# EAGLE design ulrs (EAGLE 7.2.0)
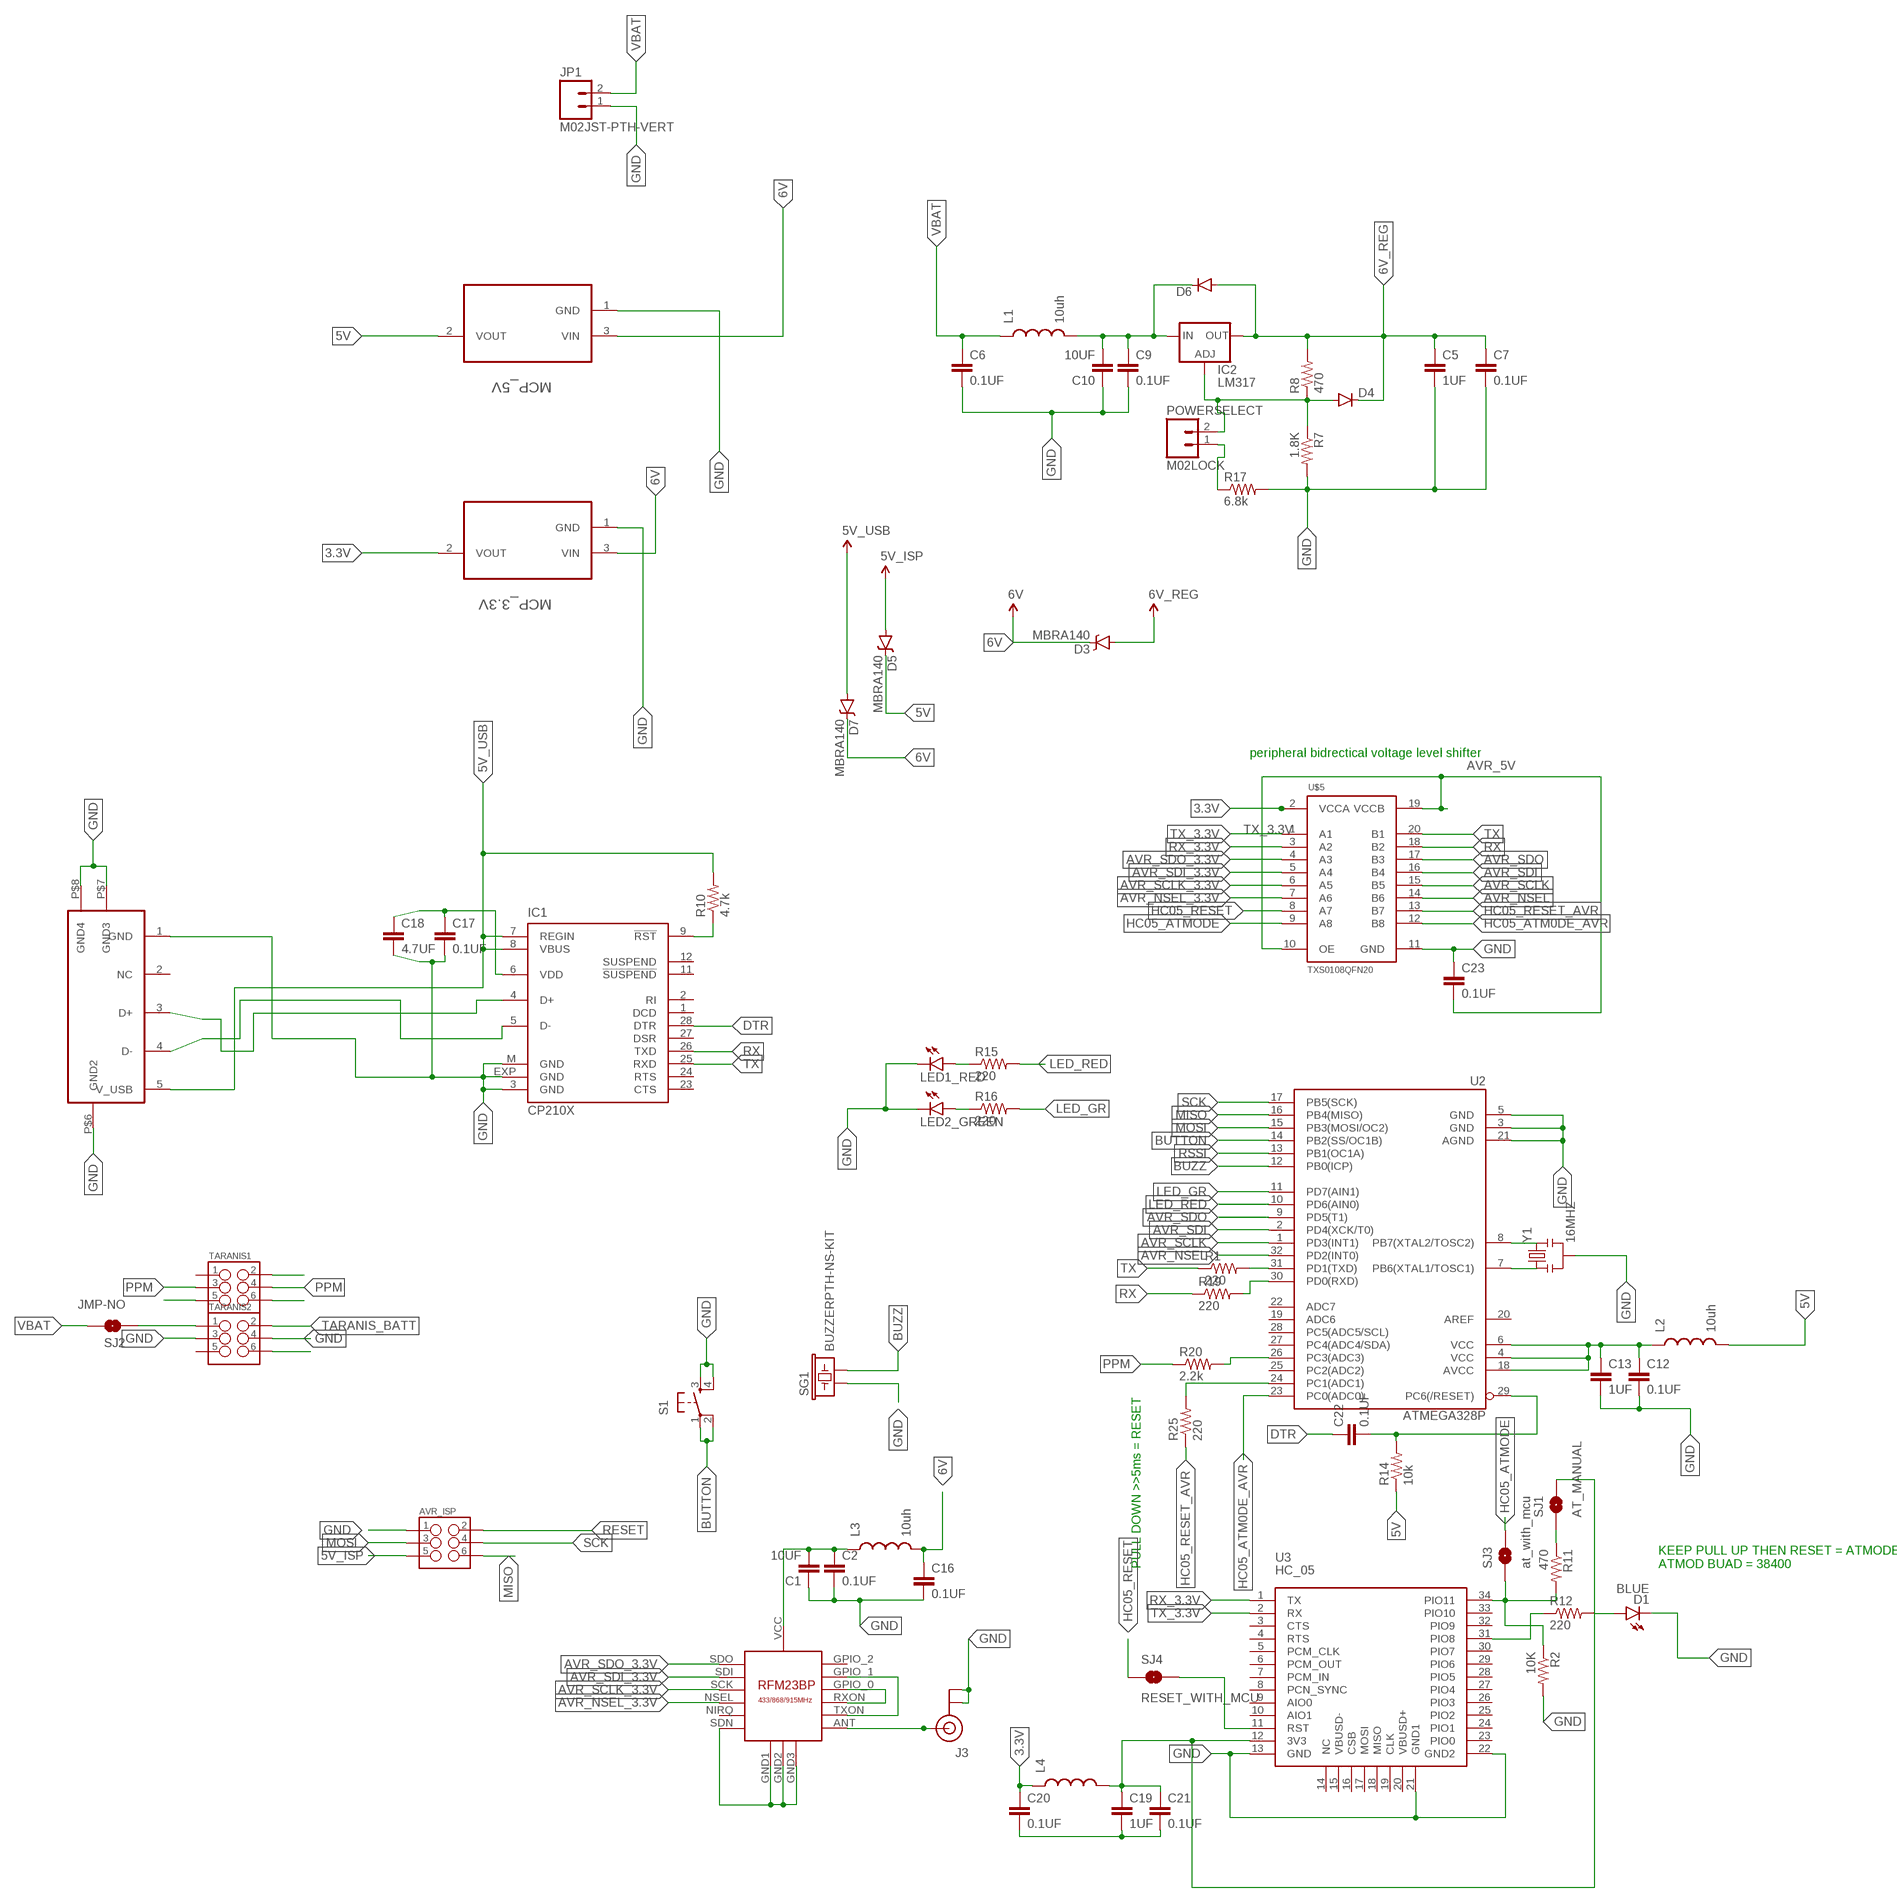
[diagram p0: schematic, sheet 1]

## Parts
AVR_ISP  M03X2FEMALE_SMD  [2X3_SMD]
C1  10UF  CAP1206  [1206]
C2  0.1UF  CAP0402-CAP  [0402-CAP]
C5  1UF  CAP0402-CAP  [0402-CAP]
C6  0.1UF  CAP0402-CAP  [0402-CAP]
C7  0.1UF  CAP0402-CAP  [0402-CAP]
C9  0.1UF  CAP0402-CAP  [0402-CAP]
C10  10UF  CAP1206  [1206]
C12  0.1UF  CAP0402-CAP  [0402-CAP]
C13  1UF  CAP0402-CAP  [0402-CAP]
C16  0.1UF  CAP0402-CAP  [0402-CAP]
C17  0.1UF  CAP0402-CAP  [0402-CAP]
C18  4.7UF  CAP0402-CAP  [0402-CAP]
C19  1UF  CAP0402-CAP  [0402-CAP]
C20  0.1UF  CAP0402-CAP  [0402-CAP]
C21  0.1UF  CAP0402-CAP  [0402-CAP]
C22  0.1UF  CAP0402-CAP  [0402-CAP]
C23  0.1UF  CAP0402-CAP  [0402-CAP]
D1  BLUE  LED-BLUE0603  [LED-0603]
D3  MBRA140  DIODE-SCHOTTKY-MBRA140  [SMA-DIODE]
D4  DIODESMA  [SMA-DIODE]
D5  MBRA140  DIODE-SCHOTTKY-MBRA140  [SMA-DIODE]
D6  DIODESMA  [SMA-DIODE]
D7  MBRA140  DIODE-SCHOTTKY-MBRA140  [SMA-DIODE]
IC1  CP210X  CP210X_USB_UART  [MLP28]
IC2  LM317  LM317MBSTT3  [SOT223]
J3  U.FL  [U.FL]
JP1  M02JST-PTH-VERT  [JST-2-PTH-VERT]
L1  10uh  INDUCTOR1007  [1007]
L2  10uh  INDUCTOR1007  [1007]
L3  10uh  INDUCTOR1007  [1007]
L4  INDUCTOR1007  [1007]
LED1_RED  LED3MM  [LED3MM]
LED2_GREEN  LED3MM  [LED3MM]
MCP_3.3V  MCP1700T-3302E/TT  [SOT95P237X112-3N]
MCP_5V  MCP1700T-5002E/TT  [SOT95P237X112-3N]
POWERSELECT  M02LOCK  [1X02_LOCK]
R1  220  RESISTOR0603-RES  [0603-RES]
R2  10K  RESISTOR0603-RES  [0603-RES]
R7  1.8K  RESISTOR0603-RES  [0603-RES]
R8  470  RESISTOR0603-RES  [0603-RES]
R10  4.7k  RESISTOR0603-RES  [0603-RES]
R11  470  RESISTOR0603-RES  [0603-RES]
R12  220  RESISTOR0603-RES  [0603-RES]
R14  10k  RESISTOR0603-RES  [0603-RES]
R15  220  RESISTOR0603-RES  [0603-RES]
R16  220  RESISTOR0603-RES  [0603-RES]
R17  6.8k  RESISTOR0603-RES  [0603-RES]
R19  220  RESISTOR0603-RES  [0603-RES]
R20  2.2k  RESISTOR0603-RES  [0603-RES]
R25  220  RESISTOR0603-RES  [0603-RES]
S1  TAC_SWITCHSMD  [TACTILE-SWITCH-SMD]
SG1  BUZZERPTH-NS-KIT  [BUZZER-12MM-NS-KIT]
SJ1  AT_MANUAL  JUMPER-PAD-2-NOYES_SILK  [PAD-JUMPER-2-NO_YES_SILK]
SJ2  JMP-NO  JUMPER-PAD-2-NOYES_SILK  [PAD-JUMPER-2-NO_YES_SILK]
SJ3  at_with_mcu  JUMPER-PAD-2-NOYES_SILK  [PAD-JUMPER-2-NO_YES_SILK]
SJ4  RESET_WITH_MCU  JUMPER-PAD-2-NOYES_SILK  [PAD-JUMPER-2-NO_YES_SILK]
TARANIS1  M03X2FEMALE_SMD  [2X3_SMD]
TARANIS2  M03X2FEMALE_SMD  [2X3_SMD]
U2  ATMEGA328P  ATMEGA328_SMT  [TQFP32-08]
U3  HC_05  [BLUETOOTH_SMD]
U$1  USB_VERTICAL_REV2  [USB_MINI_VERTICAL]
U$3  RFM23BP  [RFM23BP]
U$5  TXS0108QFN20  [QFN20-RGY]
Y1  16MHZ  RESONATOR16MHZ  [RESONATOR-SMD]

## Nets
3.3V: C20.1 L4.1 MCP_3.3V.2(VOUT) U$5.2(VCCA)
5V: D5.C L2.2 MCP_5V.2(VOUT) R14.1
5V_ISP: AVR_ISP.5 D5.A
5V_USB: D7.A IC1.7(REGIN) IC1.8(VBUS) R10.2 U$1.5(V_USB)
6V: C16.1 D3.C D7.C L3.2 MCP_3.3V.3(VIN) MCP_5V.3(VIN)
6V_REG: C5.1 C7.1 D3.A D4.C D6.A IC2.4(OUT) R8.2
AVR_5V: C12.1 C13.1 C23.2 L2.1 U2.4(VCC) U2.6(VCC) U2.18(AVCC) U$5.10(OE) U$5.19(VCCB)
AVR_NSEL: U2.32(PD2(INT0)) U$5.14(B6)
AVR_NSEL_3.3V: U$3.NSEL U$5.7(A6)
AVR_SCLK: U2.1(PD3(INT1)) U$5.15(B5)
AVR_SCLK_3.3V: U$3.SCK U$5.6(A5)
AVR_SDI: U2.2(PD4(XCK/T0)) U$5.16(B4)
AVR_SDI_3.3V: U$3.SDI U$5.5(A4)
AVR_SDO: U2.9(PD5(T1)) U$5.17(B3)
AVR_SDO_3.3V: U$3.SDO U$5.4(A3)
BUTTON: S1.1 S1.2 U2.14(PB2(SS/OC1B))
BUZZ: SG1.- U2.12(PB0(ICP))
DTR: C22.1 IC1.28(DTR)
GND: AVR_ISP.1 C1.1 C2.2 C5.2 C6.2 C7.2 C9.2 C10.1 C12.2 C13.2 C16.2 C17.2 C18.2 C19.2 C20.2 C21.2 C23.1 D1.C IC1.3(GND) IC1.EXP(GND) IC1.M(GND) J3.P$1(GND) J3.P$2(GND) JP1.1 LED1_RED.K(C) LED2_GREEN.K(C) MCP_3.3V.1(GND) MCP_5V.1(GND) R2.2 R7.2 R17.2 S1.3 S1.4 SG1.+ TARANIS2.3 TARANIS2.4 U2.3(GND) U2.5(GND) U2.21(AGND) U3.13(GND) U3.21(GND1) U3.22(GND2) U$1.1(GND) U$1.P$6(GND2) U$1.P$7(GND3) U$1.P$8(GND4) U$3.GND1 U$3.GND2 U$3.GND3 U$3.SDN U$5.11(GND) Y1.2
HC05_ATM0DE_AVR: U2.23(PC0(ADC0)) U$5.12(B8)
HC05_ATMODE: SJ3.2 U$5.9(A8)
HC05_RESET: SJ4.1 U$5.8(A7)
HC05_RESET_AVR: R25.1 U$5.13(B7)
LED_GR: R16.2 U2.11(PD7(AIN1))
LED_RED: R15.2 U2.10(PD6(AIN0))
MISO: AVR_ISP.6 U2.16(PB4(MISO))
MOSI: AVR_ISP.3 U2.15(PB3(MOSI/OC2))
N$1: C9.1 C10.2 D6.C IC2.3(IN) L1.2
N$3: D4.A IC2.1(ADJ) POWERSELECT.2 R7.1 R8.1
N$4: R11.1 SJ1.1
N$6: IC1.5(D-) U$1.4(D-)
N$7: U2.8(PB7(XTAL2/TOSC2)) Y1.3
N$8: U2.7(PB6(XTAL1/TOSC1)) Y1.1
N$9: SJ4.2 U3.11(RST)
N$10: TARANIS1.6
N$11: D1.A R12.2
N$13: IC1.4(D+) U$1.3(D+)
N$14: C1.2 C2.1 L3.1 U$3.VCC
N$15: C19.1 C21.1 L4.2 SJ1.2 U3.12(3V3)
N$17: R25.2 U2.24(PC1(ADC1))
N$18: U$3.GPIO_0 U$3.RXON
N$19: U$3.GPIO_1 U$3.TXON
N$20: TARANIS1.5
N$21: J3.P$3(SIGNAL) U$3.ANT
N$22: R2.1 R11.2 SJ3.1 U3.34(PIO11)
N$26: TARANIS1.2
N$27: POWERSELECT.1 R17.1
N$28: IC1.9(!RST) R10.1
N$29: C17.1 C18.1 IC1.6(VDD)
N$31: LED1_RED.A R15.1
N$32: R12.1 U3.31(PIO8)
N$34: LED2_GREEN.A R16.1
N$35: R1.2 U2.31(PD1(TXD))
N$38: R20.2 U2.26(PC3(ADC3))
N$42: TARANIS2.6
N$43: R19.2 U2.30(PD0(RXD))
PPM: R20.1 TARANIS1.3 TARANIS1.4
RESET: AVR_ISP.2 C22.2 R14.2 U2.29(PC6(/RESET))
RSSI: U2.13(PB1(OC1A))
RX: IC1.26(TXD) R19.1 U$5.18(B2)
RX_3.3V: U3.1(TX) U$5.3(A2)
SCK: AVR_ISP.4 U2.17(PB5(SCK))
TARANIS_BATT: SJ2.1 TARANIS2.1 TARANIS2.2
TX: IC1.25(RXD) R1.1 U$5.20(B1)
TX_3.3V: U3.2(RX) U$5.1(A1)
VBAT: C6.1 JP1.2 L1.1 SJ2.2
Unconnected: IC1.1(DCD) IC1.2(RI) IC1.11(!SUSPEND) IC1.12(SUSPEND) IC1.23(CTS) IC1.24(RTS) IC1.27(DSR) TARANIS1.1 TARANIS2.5 U2.19(ADC6) U2.20(AREF) U2.22(ADC7) U2.25(PC2(ADC2)) U2.27(PC4(ADC4/SDA)) U2.28(PC5(ADC5/SCL)) U3.3(CTS) U3.4(RTS) U3.5(PCM_CLK) U3.6(PCM_OUT) U3.7(PCM_IN) U3.8(PCN_SYNC) U3.9(AIO0) U3.10(AIO1) U3.14(NC) U3.15(VBUSD-) U3.16(CSB) U3.17(MOSI) U3.18(MISO) U3.19(CLK) U3.20(VBUSD+) U3.23(PIO0) U3.24(PIO1) U3.25(PIO2) U3.26(PIO3) U3.27(PIO4) U3.28(PIO5) U3.29(PIO6) U3.30(PIO7) U3.32(PIO9) U3.33(PIO10) U$1.2(NC) U$3.GPIO_2 U$3.NIRQ

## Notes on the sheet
- peripheral bidrectical voltage level shifter
- PULL DOWN >>5ms = RESET
- KEEP PULL UP THEN RESET = ATMODE
  ATMOD BUAD = 38400

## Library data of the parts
AVR_ISP TARANIS1 TARANIS2 = SparkFun-Connectors:M03X2: 2x3 .1" header. Shrouded, with keying- CONN-10681 SMT- CONN-11415 Pogo pins- HW-11044; PROD_ID: CONN-11290
C1 C10 = SparkFun-Capacitors:CAP: Capacitor
C2 C5-C7 C9 C12 C13 C16-C23 = SparkFun-Passives:CAP: Capacitor
D1 = SparkFun-LED:LED-BLUE: Blue LEDs for production use; PROD_ID: DIO-08575
D3 D5 D7 = SparkFun-DiscreteSemi:DIODE-SCHOTTKY: Schottky diodes in SFE's production catalog; PROD_ID: DIO-08053
D4 D6 = SparkFun-DiscreteSemi:DIODE: Diode
IC1 = SparkFun-DigitalIC:CP210X_USB_UART: Single-Chip USB to UART Bridge Source: www.silabs.com .. CP2101.pdf / cp2102.pdf. Spark Fun Electronics SKU : COM-00310
IC2 = v-reg:LM317?*: 500 mA Adjustable Output Positive Voltage Regulator Source: http://www.onsemi.co.jp .. LM317M-D.PDF
J3 = SparkFun-Connectors:U.FL: SMD antenna connector- WRL-09144; PROD_ID: CONN-09193
JP1 POWERSELECT = SparkFun-Connectors:M02: Standard 2-pin 0.1" header. Use with
L1-L4 = SparkFun-Passives:INDUCTOR: Inductors
LED1_RED LED2_GREEN = SparkFun-LED:LED: LEDs
MCP_3.3V = Microchip_By_element14_Batch_1:MCP1700T-3302E/TT: Low Quiescent Current LDO; MPN: MCP1700T-3302E/TT; OC_FARNELL: 1296592; OC_NEWARK: 88H9817; PACKAGE: SOT23-3; SUPPLIER: Microchip
MCP_5V = Microchip_By_element14_Batch_1:MCP1700T-5002E/TT: Low Quiescent Current LDO; MPN: MCP1700T-5002E/TT; OC_FARNELL: 1296593; OC_NEWARK: 88H9819; PACKAGE: SOT23-3; SUPPLIER: Microchip
R1 R2 R7 R8 R10-R12 R14-R17 R19 R20 R25 = SparkFun-Resistors:RESISTOR: Resistor
S1 = SparkFun-Electromechanical:TAC_SWITCH: Momentary Switch Button commonly used for reset or general input. Spark Fun Electronics SKU : COM-00097 SMT- SWCH-08247
SG1 = SparkFun-Electromechanical:BUZZER: Buzzer 12mm; PROD_ID: COMP-08253
SJ1-SJ4 = SparkFun-Passives:JUMPER-PAD-2-NO
U2 = SparkFun-DigitalIC:ATMEGA328_SMT: 32-Pin Atmega328 part Commonly used on Arduino compatible boards Available in QFP and QFN packages TQFP is IC-09069 QFN is non-stock; PROD_ID: IC-09069
U3 = Bluetooth HC-05:HC_05: HC-05 Bluetooth Module
U$1 = SparkFun-Connectors:USB_VERTICAL_REV2
U$3 = RFM23BP:RFM23BP: HopeRF RFM23BP Library by: http://projects.weber-itam.de
U$5 = pixhawk2:TXS0108
Y1 = SparkFun-FreqCtrl:RESONATOR: Resonator Small SMD resonator. Used, eg, on the Arduino Pro/ Pro Mini boards. 8MHz- XTAL-08895 16MHz- XTAL-08900; PROD_ID: XTAL-08900

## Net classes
0 signal: width 0.15 mm, drill 0.15 mm, clearance 0.152 mm
1 power: width 0.15 mm, drill 0.2 mm, clearance 0.152 mm

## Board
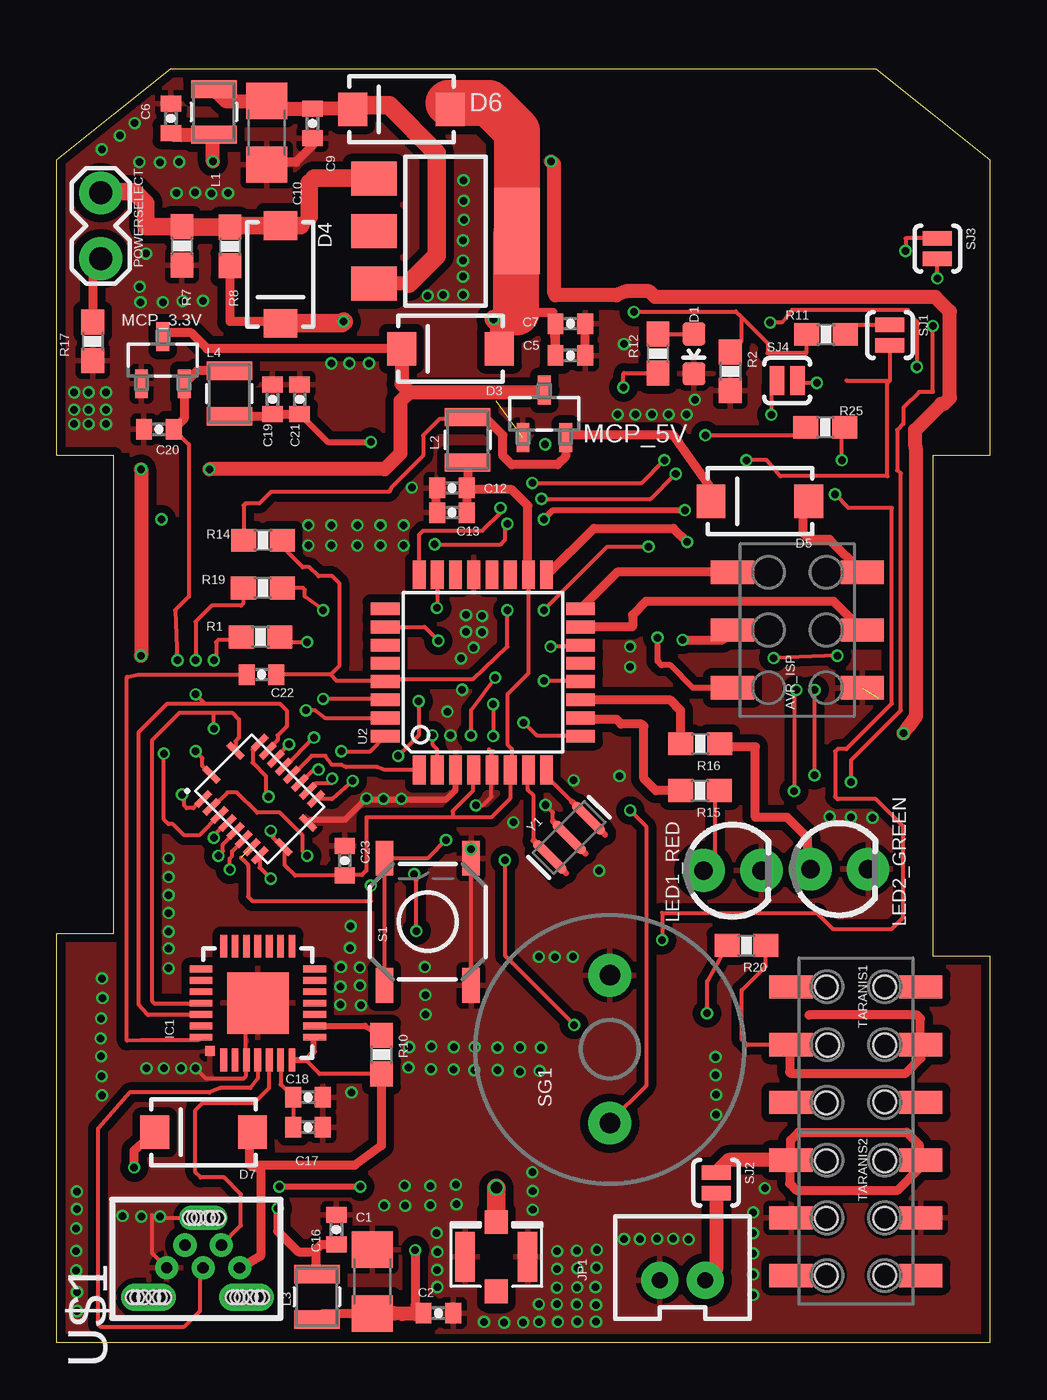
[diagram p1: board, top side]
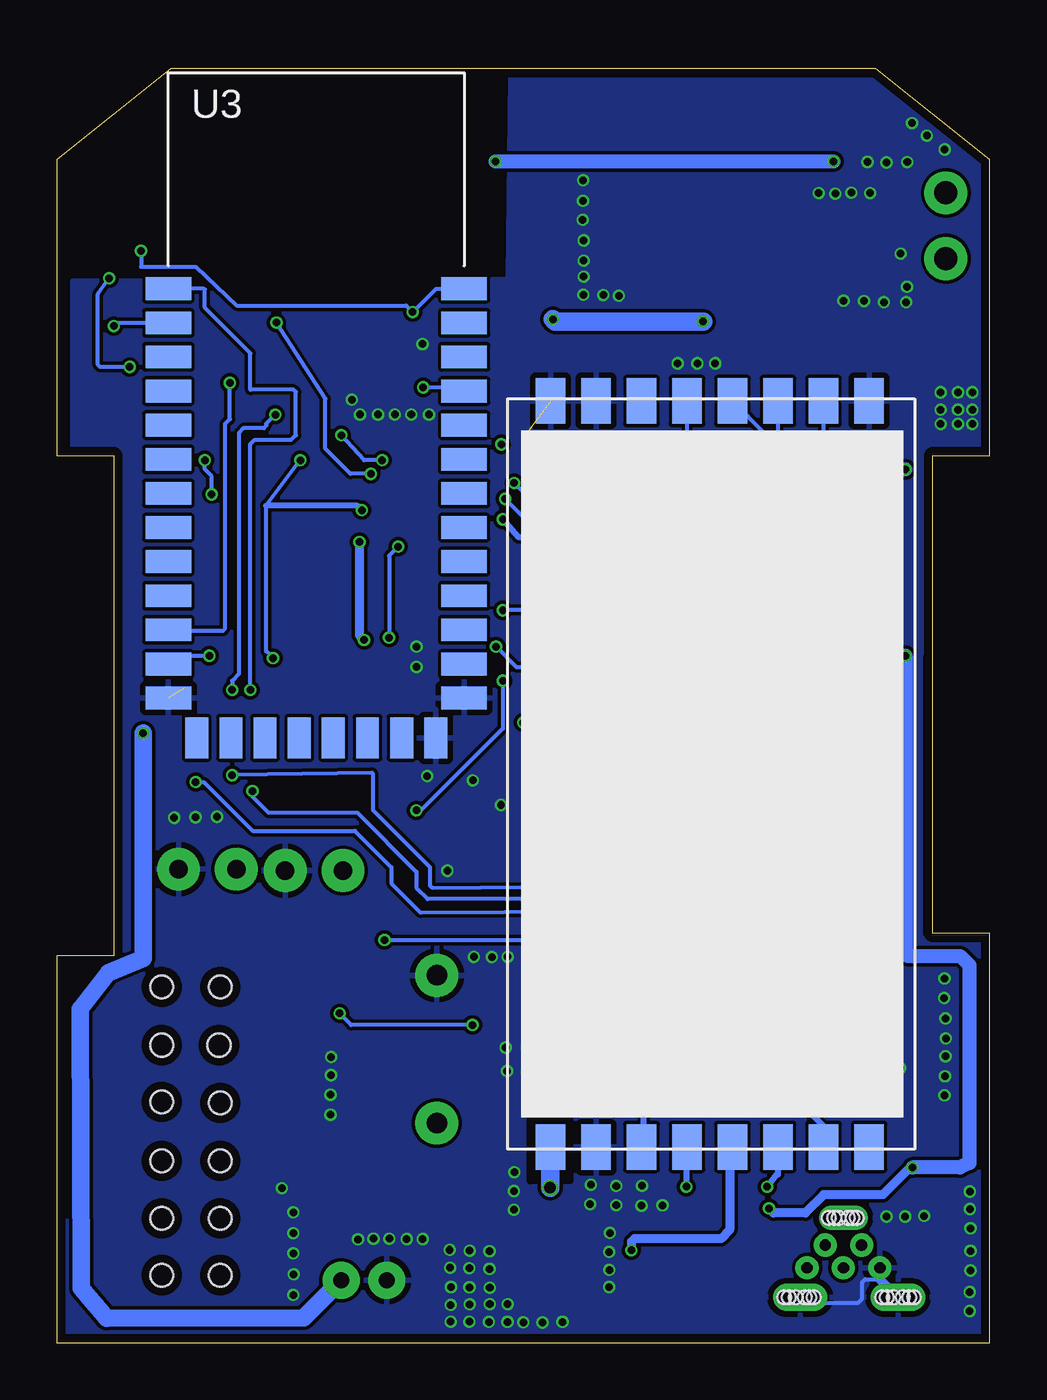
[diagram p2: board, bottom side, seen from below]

Size 41 x 56 mm. Coordinates in mm from the lower left corner, seen from the top.
Outline: 0,18 2.5,18 2.5,39 0,39 0,52 5,56 36,56 41,52 41,39 38.5,39 38.5,17 41,17 41,0 0,0 0,18
Copper layers (1*16): Top 0.0356mm / dielectric 1.5011mm / Bottom 0.0356mm
Design rules "oshpark-2layer *": minimum track width 6mil, minimum drill 13mil, track to track 6mil, track to pad 6mil, pad to pad 6mil, via to via 6mil, smd to smd 6mil, copper to edge 15mil, drill to drill 6mil, minimum pad ring 4mil, minimum via ring 4mil, stop-mask expansion 2mil, vias tented up to drill 13mil, thermal gap 10mil
Holes 1 mm at 33.83,15.64 36.39,15.64 33.88,13.08 36.39,13.08 33.83,10.54 36.39,10.59 33.83,8 36.39,8 33.83,5.46 36.39,5.46 36.39,2.97 33.83,2.97
tRestrict: area 18.9,1.6 to 19.7,4.7; area 21.5,20.3 to 24.2,23; area 20.9,21 to 23.6,23.7
bRestrict: area 18.4,7.1 to 19.2,10.1; area 18.9,7.1 to 19.7,10.1; area 19.4,7.1 to 20.2,10.1

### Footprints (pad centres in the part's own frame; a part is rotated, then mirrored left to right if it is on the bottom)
2X3_SMD = smd 1.02 x 1.9: 1 -2.54,-2.85; 2 -2.54,2.85; 3 0,-2.85; 4 0,2.85; 5 2.54,-2.85; 6 2.54,2.85
1206 = smd 1.6 x 1.8: 1 -1.4,0; 2 1.4,0
0402-CAP = smd 0.7 x 0.9: 1 -0.65,0; 2 0.65,0
LED-0603 = smd 1 x 1: A 0,-0.877; C 0,0.877
SMA-DIODE = smd 1.27 x 1.47: A -2.15,0; C 2.15,0
MLP28 = smd 1 x 0.3: 1 -2.5,1.5; 2 -2.5,1; 3 -2.5,0.5; 4 -2.5,0; 5 -2.5,-0.5; 6 -2.5,-1; 7 -2.5,-1.5; 15 2.5,-1.5; 16 2.5,-1; 17 2.5,-0.5; 18 2.5,0; 19 2.5,0.5; 20 2.5,1; 21 2.5,1.5 | smd 0.3 x 1: 8 -1.5,-2.5; 9 -1,-2.5; 10 -0.5,-2.5; 11 0,-2.5; 12 0.5,-2.5; 13 1,-2.5; 14 1.5,-2.5; 22 1.5,2.5; 23 1,2.5; 24 0.5,2.5; 25 0,2.5; 26 -0.5,2.5; 27 -1,2.5; 28 -1.5,2.5 | smd 2.7 x 2.7: EXP 0,0 | smd 0.435 x 0.435: M -2.103,2.103
SOT223 = smd 1.5 x 2: 1 -2.3,-3.15; 2 0,-3.15; 3 2.3,-3.15 | smd 3.8 x 2: 4 0,3.15
U.FL = smd 2.2 x 0.85: P$1 0,1.375; P$2 0,-1.375 | smd 1.05 x 1: P$3 1.525,0; P$4 -1.525,0
JST-2-PTH-VERT = drill 0.7 pad 1.626: 1 -1,-0.55; 2 1,-0.55
1007 = smd 2 x 0.8: 1 0,1; 2 0,-1
LED3MM = drill 0.813 pad 1.88: A -1.27,0; K 1.27,0
SOT95P237X112-3N = smd 0.559 x 1.27: 1 -0.94,-1.041; 2 0.94,-1.041; 3 0,1.041
1X02_LOCK = drill 1.016 pad 1.88: 1 -0.178,0; 2 2.718,0
0603-RES = smd 1.1 x 1: 1 -0.85,0; 2 0.85,0
TACTILE-SWITCH-SMD = smd 1.524 x 0.762: 1 -2.794,1.905; 2 2.794,1.905; 3 -2.794,-1.905; 4 2.794,-1.905
BUZZER-12MM-NS-KIT = drill 0.9 pad 1.88: + 3.25,0; - -3.25,0
PAD-JUMPER-2-NO_YES_SILK = smd 0.635 x 1.27: 1 -0.45,0; 2 0.45,0
TQFP32-08 = smd 1.27 x 0.559: 1 -4.293,2.8; 2 -4.293,2; 3 -4.293,1.2; 4 -4.293,0.4; 5 -4.293,-0.4; 6 -4.293,-1.2; 7 -4.293,-2; 8 -4.293,-2.8; 17 4.293,-2.8; 18 4.293,-2; 19 4.293,-1.2; 20 4.293,-0.4; 21 4.293,0.4; 22 4.293,1.2; 23 4.293,2; 24 4.293,2.8 | smd 0.559 x 1.27: 9 -2.8,-4.293; 10 -2,-4.293; 11 -1.2,-4.293; 12 -0.4,-4.293; 13 0.4,-4.293; 14 1.2,-4.293; 15 2,-4.293; 16 2.8,-4.293; 25 2.8,4.293; 26 2,4.293; 27 1.2,4.293; 28 0.4,4.293; 29 -0.4,4.293; 30 -1.2,4.293; 31 -2,4.293; 32 -2.8,4.293
BLUETOOTH_SMD = smd 2 x 1: 1 -6.35,3.81; 2 -6.35,2.31; 3 -6.35,0.81; 4 -6.35,-0.69; 5 -6.35,-2.19; 6 -6.35,-3.69; 7 -6.35,-5.19; 8 -6.35,-6.69; 9 -6.35,-8.19; 10 -6.35,-9.69; 11 -6.35,-11.19; 12 -6.35,-12.69; 13 -6.35,-14.19; 22 6.65,-14.19; 23 6.65,-12.69; 24 6.65,-11.19; 25 6.65,-9.69; 26 6.65,-8.19; 27 6.65,-6.69; 28 6.65,-5.19; 29 6.65,-3.69; 30 6.65,-2.19; 31 6.65,-0.69; 32 6.65,0.81; 33 6.65,2.31; 34 6.65,3.81 | smd 1 x 1.8: 14 -5.1,-15.94; 15 -3.6,-15.94; 16 -2.1,-15.94; 17 -0.6,-15.94; 18 0.9,-15.94; 19 2.4,-15.94; 20 3.9,-15.94; 21 5.4,-15.94
USB_MINI_VERTICAL = drill 0.5 pad 1.016: 1 -0.8,2.6; 2 0.2,1.8; 3 -0.8,1; 4 0.2,0.2; 5 -0.8,-0.6 | drill 0.6 pad 1.2 long: P$6 -2.1,-0.9; P$7 -2.1,3.4 | drill 0.6 pad 1.067 long: P$8 1.4,1 | hole 0.6: -2.1,3.2; -2.1,2.9; -2.1,3.6; -2.1,3.9; -2.1,2.7; -2.1,4.1; -2.1,-0.7; -2.1,-0.5; -2.1,-0.3; -2.1,-1.1; -2.1,-1.4; -2.1,-1.6; 1.4,0.8; 1.4,0.6; 1.4,1.2; 1.4,1.4; 1.4,0.6; 1.4,0.346; 1.4,1.591
RFM23BP = smd 2 x 1.3: ANT 16.9,-7.5; GND1 -15.9,6.5; GND2 -15.9,-7.5; GND3 16.9,-5.5; GPIO_0 16.9,2.5; GPIO_1 16.9,4.5; GPIO_2 16.9,6.5; NIRQ -15.9,-3.5; NSEL -15.9,-1.5; RXON 16.9,-1.5; SCK -15.9,0.5; SDI -15.9,2.5; SDN -15.9,-5.5; SDO -15.9,4.5; TXON 16.9,-3.5; VCC 16.9,0.5
QFN20-RGY = smd 0.28 x 0.85: 1 -0.75,2.25; 10 -0.75,-2.25; 11 0.75,-2.25; 20 0.75,2.25 | smd 0.85 x 0.28: 2 -1.75,1.75; 3 -1.75,1.25; 4 -1.75,0.75; 5 -1.75,0.25; 6 -1.75,-0.25; 7 -1.75,-0.75; 8 -1.75,-1.25; 9 -1.75,-1.75; 12 1.75,-1.75; 13 1.75,-1.25; 14 1.75,-0.75; 15 1.75,-0.25; 16 1.75,0.25; 17 1.75,0.75; 18 1.75,1.25; 19 1.75,1.75
RESONATOR-SMD = smd 0.45 x 1.905: 1 -1.2,0; 2 0,0; 3 1.2,0

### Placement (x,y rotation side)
AVR_ISP  32.54,31.33 90 top
C1  13.87,2.69 270 top
C2  16.76,1.3 0 top
C5  22.57,43.4 0 top
C6  5.01,53.83 90 top
C7  22.57,44.8 0 top
C9  11.23,53.6 270 top
C10  9.22,53.19 90 top
C12  17.37,37.57 180 top
C13  17.37,36.49 180 top
C16  12.29,4.97 90 top
C17  11.04,9.47 0 top
C18  11.04,10.79 0 top
C19  9.48,41.48 90 top
C20  4.48,40.16 180 top
C21  10.67,41.48 90 top
C22  9,29.37 0 top
C23  12.65,21.19 270 top
D1  27.99,43.47 180 top
D3  17.3,43.7 180 top
D4  9.83,46.97 270 top
D5  30.9,37 180 top
D6  15.15,54.22 180 top
D7  6.45,9.25 180 top
IC1  8.83,14.93 90 top
IC2  17.08,48.87 270 top
J3  19.31,3.77 90 top
JP1  27.5,3.3 0 top
L1  6.9,54.11 180 top
L2  18.05,39.69 180 top
L3  11.43,2.01 180 top
L4  7.58,41.73 0 top
LED1_RED  29.69,20.76 0 top
LED2_GREEN  34.38,20.82 0 top
MCP_3.3V  4.66,43.2 0 top
MCP_5V  21.42,40.83 0 top
POWERSELECT  1.93,47.84 90 top
R1  8.95,31.02 0 top
R2  29.6,42.7 270 top
R7  5.5,48.22 270 top
R8  7.61,48.19 270 top
R10  14.26,12.66 270 top
R11  33.8,44.33 180 top
R12  26.42,43.48 90 top
R14  9.06,35.28 0 top
R15  28.27,24.27 180 top
R16  28.28,26.33 180 top
R17  1.58,44.02 270 top
R19  9.05,33.18 0 top
R20  30.31,17.47 180 top
R25  33.77,40.24 180 top
S1  16.3,18.5 90 top
SG1  24.3,12.9 90 top
SJ1  36.61,44.3 270 top
SJ2  28.98,7.03 270 top
SJ3  38.7,48.1 270 top
SJ4  32.1,42.3 0 top
TARANIS1  35.12,13.11 270 top
TARANIS2  35.12,5.49 270 top
U2  18.72,29.47 90 top
U3  29.75,42.53 0 bottom
U$1  7.43,4.09 90 top
U$3  11.8,25.5 270 bottom
U$5  8.91,23.91 45 top
Y1  22.52,22.21 45 top

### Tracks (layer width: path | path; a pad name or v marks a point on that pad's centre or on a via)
3.3V  (via drill 0.33 pad 0.25)
  Top 0.178: C20.1 5.8,39.49 5.8,32.8 5.2,32.2 v5.3,30 | U$5.2 6.39,23.91 6.39,23.89 6,23.5 5.7,23.5 5.6,23.6 5.6,24 v5.5,24.1
  Top 0.406: L4.1 6.17,42.73 MCP_3.3V.2 5.59,40.62 C20.1
  Bottom 0.178: v5.5,24.1 5.5,25.1 5.3,25.4 v5.3,30
5V
  Top 0.178: R14.1 8.21,36.8 8.3,36.9 8.9,36.9 9.4,37.4 14.6,37.4 14.7,37.6 16.1,39 16.1,39.9 16.8,40.6 17.97,40.6 L2.2
  Top 0.406: L2.2 18.14,40.6 18.9,40.6 19.6,39.9 19.6,39 20,38.6 22,38.6 22.36,38.96 MCP_5V.2 22.47,39.9 27.1,39.9 28.75,37.55 D5.C
5V_ISP
  Top 0.406: AVR_ISP.5 33.95,35.31 33.09,35.31 32.8,35.6 32.8,36.75 D5.A
5V_USB
  Top 0.178: R10.2 11.55,11.81 10.93,12.43
  Top 0.254: IC1.7 10.93,12.43 11.3,12.8 11.3,13.4 IC1.8
  Top 0.406: 8.85,9.4 D7.A 8.48,9.13 8.48,7.81 | R10.2 14.26,8.66 13.1,7.8 8.79,7.8 8.48,7.81 | 8.48,7.81 8.95,7.6 8.95,3.81 8.09,3.29 U$1.5
6V  (via drill 0.33 pad 0.25, 0.33 pad 0.41)
  Top 0.406: D3.C 6.6,43.7 5.9,44.4 4.82,44.4 MCP_3.3V.3 | 9.67,5.99 v9.7,5.9 9.7,4.9 10.6,4 11.3,4 11.4,4.1 | v3.4,7.7 3.4,8.45 D7.C | L3.2 11.4,3.04 11.4,4.1 | 11.4,4.1 11.62,4.32 C16.1
  Top 0.61: D3.C 15.15,42.15 15.5,41.8 | 15.5,41.8 21.35,41.8 MCP_5V.3 | 15.5,41.8 15.1,41.4 15.1,39.1 14.4,38.4 v6.7,38.4 | v3.7,38.4 v3.7,30.2
  Bottom 0.406: v3.4,7.7 3.5,7.7 4.7,6.5 7.3,6.5 8.1,5.7 9.5,5.7 v9.7,5.9
  Bottom 0.61: v6.7,38.4 v3.7,38.4 | v3.7,30.2 3.7,17.3 3.6,17 1.3,17 0.9,16.6 0.9,7.9 1.3,7.7 v3.4,7.7
6V_REG  (via drill 0.33 pad 0.25)
  Top 0.406: 20.2,45.3 21.8,45.3 C5.1 C7.1 | 9.81,44.8 9.71,44.9 7.6,44.9 7.61,44.91 R8.2
  Top 0.813: 17.22,54.5 D6.A | 9.81,44.8 D4.C 12.52,44.81 v12.6,44.9 | 20.2,45.3 19.9,45 v19.2,45 19.45,44.75 D3.A | 20.2,48.84 IC2.4
  Top 2.032: IC2.4 20.23,53.27 19,54.5 17.22,54.5 | 20.2,45.3 20.2,48.84
  Bottom 0.813: v12.6,44.9 19.1,44.9 v19.2,45
AVR_5V  (via drill 0.33 pad 0.25)
  Top 0.178: U2.18 20.72,29.42 19.8,28.5 19.8,26.3 20,26.1 20,25.25 U2.6 19.92,23.92 19.1,23.1 17.4,23.1 | 17.4,23.1 13.6,23.1 13.6,20.76 13.4,20.56 12.67,20.56 C23.2 10.47,20.54 10.02,20.99 10.02,21.74 U$5.10 9.91,21.79 9.5,22.2 9.5,22.4 v9.4,22.5 | U$5.19 8.6,26.07 8.6,25.5 9.2,24.9 9.2,24.1 v9.3,24 | 18.3,25.15 18.29,25.14 18.29,24.26 17.4,23.37 17.4,23.1
  Top 0.254: U2.4 18.3,25.15
  Top 0.406: U2.18 20.7,33.78 20.7,36.8 20,37.5 18.09,37.5 C12.1 | L2.1 18.05,37.61 C12.1 | C12.1 18.02,36.59 C13.1
  Bottom 0.178: v9.4,22.5 9.3,22.6 v9.3,24
AVR_NSEL  (via drill 0.33 pad 0.41)
  Top 0.178: U$5.14 10.71,24.61 11.3,25.2 v11.5,25.2 | v12.5,26 13.76,26 U2.32
  Bottom 0.178: v11.5,25.2 11.7,25.4 11.7,25.6 12.1,26 v12.5,26
AVR_NSEL_3.3V  (via drill 0.33 pad 0.25)
  Top 0.178: v7.6,20.8 7.6,21.3 7.7,21.4 7.7,21.6 8.21,22.11 U$5.7
  Bottom 0.178: v7.6,20.8 8.1,21.2 8.1,22.2 8.6,22.7 8.6,34.3 10.4,36.1 10.4,39.2 10.6,39.4 12.8,39.4 13.3,39.9 U$3.NSEL
AVR_SCLK
  Top 0.178: U$5.15 10.37,24.97 11.2,25.8 11.8,25.8 12.1,25.4 12.5,25.4 12.7,25.3 14.1,25.3 14.4,25.2 15.9,25.2 U2.1
AVR_SCLK_3.3V  (via drill 0.33 pad 0.25)
  Top 0.178: v7.1,21.4 7.3,21.6 7.3,21.9 7.85,22.45 U$5.6
  Bottom 0.178: U$3.SCK 9.9,40 9.9,36.3 8,34.6 8,23 7.7,22.5 7.7,21.8 7.3,21.4 v7.1,21.4
AVR_SDI  (via drill 0.33 pad 0.41)
  Top 0.178: U$5.16 10.02,25.32 v11.3,26.6 | v16.5,26.7 16.5,26.3 16.7,26.1 16.7,25.2 U2.2
  Bottom 0.178: v11.3,26.6 16.2,26.6 v16.5,26.7
AVR_SDI_3.3V  (via drill 0.33 pad 0.25)
  Top 0.178: U$5.5 7.6,22.95 7.6,23 6.9,22.3 v6.9,22.2
  Bottom 0.178: v6.9,22.2 7.5,23.3 7.5,34.8 9.3,36.6 U$3.SDI
AVR_SDO  (via drill 0.33 pad 0.41)
  Top 0.178: U$5.17 9.62,25.72 v10.2,26.3 | v20.51,27.26 21.1,26.7 22.98,26.7 U2.9
  Bottom 0.178: v10.2,26.3 11.21,27.26 v20.51,27.26
AVR_SDO_3.3V  (via drill 0.33 pad 0.25)
  Top 0.178: U$5.4 6.25,22.3 5.6,22.3 5.1,22.8 4.9,22.8 4.7,23 v4.7,25.9
  Bottom 0.178: U$3.SDO 7.3,37.1 7.2,37 5.8,37 v4.6,36.2 4.6,26 v4.7,25.9
BUTTON  (via drill 0.33 pad 0.25)
  Top 0.178: U2.14 22.95,30.6 v21.7,30.6 | v19.26,29.24 18.2,27.8 v18.2,26.7 | v17.1,22.1 16.29,21.29 S1.2 S1.1
  Bottom 0.178: v21.7,30.6 20.8,29.7 19.72,29.7 v19.26,29.24 | v18.2,26.7 17.1,25.6 v17.1,22.1
BUZZ  (via drill 0.33 pad 0.25)
  Top 0.178: U2.12 22.98,29.1 v21.4,29.1 | v25.2,23.4 25.9,22.7 25.9,11.3 24.3,9.7 SG1.-
  Bottom 0.178: v21.4,29.1 21.4,27 25,23.4 v25.2,23.4
DTR
  Top 0.178: IC1.28 6.2,13.3 3.7,13.3 3.07,13.27 3.07,29.27 3.57,29.37 C22.1
GND  (via drill 0.33, 0.33 pad 0.25)  (2 unrouted)
  Top 0.178: C1.1 14.27,4.53 | 12.37,5.7 C16.2 | IC1.3 8.3,12.46 | 8.3,12.46 8.3,13.9 8.83,14.43 IC1.EXP | S1.3 S1.4 | 8.3,12.46 8.3,11.7 8.2,11.6 6.56,11.6 v6.1,12.06 | v18.41,23.62 18.72,23.62 19.1,24 19.1,25.9 19.2,26 19.1,26 19,26.1 | 21.8,22.93 21.8,23.32 v21.48,23.64 | U$1.1 4.19,3.93 4.19,5.6 4.3,5.49 U$1.P$8
  Top 0.254: 17.53,25.26 17.53,24.28 17.49,24.24 17.46,24.24 17.11,23.89 13.65,23.89 v13.61,23.93 12.68,23 11.19,23 U$5.11
  Top 0.406: C9.2 11.23,52.63 10.5,51.9 9.33,51.9 C10.1 | C5.2 C7.2 | C13.2 16.62,37.48 C12.2
  Bottom 0.178: U$1.P$6 8.1,1.76 5.78,1.76 5.61,1.93 5.61,2.65 5.47,2.79 4.83,2.79
  Bottom 0.406: U$1.P$7 4.83,2.79 U$1.1
  other vias: 3.94,12.06 4.7,12.06 5.46,12.06 12.95,11 12.06,43.05 12.85,43.05 13.72,43.05 0.76,41.78 1.4,41.78 1.4,41.02 1.4,40.39 0.76,40.39 2.16,41.78 2.16,41.02 2.16,40.39 0.76,41.02 15.24,35.94 11.05,35.94 12.06,35.94 11.05,35.05 12.06,35.05 13.21,35.05 13.21,35.94 14.22,35.94 14.22,35.05 15.24,35.05 24.64,40.81 25.43,40.81 26.15,40.81 26.89,40.81 27.68,40.81 17.3,26.7 18.2,21.7 15.6,37.6 20.06,22.88 17.16,27.75 7.52,50.54 6.79,50.52 6.08,50.56 5.26,50.54 18.69,31.95 17.98,31.99 17.98,31.25 18.68,31.24 18.31,30.56 17.76,30.08 17.81,28.71 27.77,4.54 27.09,4.57 26.39,4.57 25.62,4.55 24.93,4.55 23.7,0.92 22.88,0.92 22.02,0.91 21.2,0.91 20.5,0.89 19.66,0.88 18.77,0.91 23.7,1.66 22.86,1.68 21.98,1.69 21.18,1.69 21.98,2.41 22.86,2.43 23.68,2.44 23.71,3.29 22.88,3.27 21.98,3.24 21.98,4.02 22.86,4.04 23.73,4.08 28.95,12.56 28.95,11.76 28.98,10.9 28.98,10.02 1.99,16.01 2,15.15 1.95,14.25 1.93,13.37 1.95,12.59 1.97,11.71 1.99,10.87 6.42,45.81 5.53,45.79 4.66,45.74 3.67,45.74 3.63,46.42 3.92,47.88 5.38,51.91 4.54,51.89 3.62,51.9 14.36,23.91 15.14,23.91 20.89,7.49 20.91,6.66 20.91,5.84 17.54,6.94 17.57,6.08 16.41,6.89 16.41,6.04 4.54,5.54 3.71,5.54 2.88,5.57 0.88,6.64 0.88,5.87 0.84,5.02 0.84,4.03 0.84,3.17 0.89,2.22 0.89,1.39 21.27,12.97 20.36,12.98 19.36,12.97 18.36,13 17.45,12.99 16.45,13.02 15.48,12.99 15.46,12.1 16.45,12.02 17.43,12.01 18.34,11.98 19.38,11.98 20.34,11.91 21.27,12.97 21.21,11.94 21.18,16.96 21.89,16.95 22.68,16.96 23.84,20.75 24.73,24.91 22.71,24.72 35.84,23.08 34.91,23.1 33.97,23.12 28.04,41.46 24.93,43.91 3.42,53.62 2.77,53.07 1.98,52.46 17.87,51.1 17.88,50.2 17.89,49.37 17.85,48.46 17.85,47.57 17.85,46.87 17.86,46.07 16.98,46.06 16.3,46.03 4.92,16.46 4.92,17.33 4.92,18.07 4.92,18.89 4.92,19.67 4.92,20.47 4.92,21.29 31.11,6.79 30.61,5.72 30.61,4.81 30.61,3.92 30.59,3 30.61,2.1 25.2,30.6 25.2,29.71 15.29,6.9 15.3,6.02 14.38,6.03 16.7,4.82 16.73,3.99 16.71,3.2 16.73,2.44 13.37,14.83 12.46,14.85 12.46,15.65 13.32,15.7 13.31,16.49 12.48,16.51 12.88,17.35 12.91,18.31 16.18,16.51 16.2,15.28 16.2,14.43
  pour Top (isolate 0.356): 40.7,0.2 0.3,0.3 0.2,17.6 3.1,17.7 3.3,39.2 0.1,39.2 0.1,51.8 5,55.8 35.9,55.8 40.8,51.9 40.8,39.2 38,39.2 37.8,39.2 37.7,16.7 40.7,16.7 40.8,0.5
  pour Bottom (isolate 0.127): 40.6,0.25 40.4,0.45 0.3,0.45 0.25,0.5 0.25,17.55 0.3,17.6 2.75,17.6 3,17.85 3,39.1 2.7,39.4 0.35,39.4 0.3,39.45 0.3,51.65 5.02,55.54 21.1,55.68 21.2,46.78 40.34,46.69 40.35,39.36 38.31,39.35 38.14,16.98 38.12,16.77 40.69,16.75 40.82,0.35 40.59,0.19
  pour Bottom (isolate 0.356): 40.46,-0.56 40.26,-0.36 0.16,-0.36 0.11,-0.31 0.11,16.74 0.16,16.79 2.61,16.79 2.86,17.04 2.86,38.29 2.56,38.59 0.21,38.59 0.16,38.64 0.16,50.84 4.88,54.73 18.05,54.67 18.19,46.33 40.33,46.48 40.21,38.55 38.17,38.54 38,16.17 37.98,15.96 40.55,15.94 40.68,-0.46 40.45,-0.62
HC05_ATM0DE_AVR  (via drill 0.33)
  Top 0.178: U2.23 16.72,32.32 v16.7,32.3 | v15.9,28.2 15.9,26.7 v15,25.8 | v13,24.7 12.1,23.9 U$5.12
  Bottom 0.178: v16.7,32.3 16.4,32.3 16.1,32 16.1,28.4 v15.9,28.2 | v15,25.8 14,25.8 v13,24.7
HC05_ATMODE  (via drill 0.33, 0.33 pad 0.25)
  Top 0.178: v21.3,37.1 26.1,37.1 v27.2,38.2 | v19.8,36 19.7,35.9 19.7,35.3 19.5,35.1 16.7,35.1 16.62,35.08 v16.6,35.1 | v31.35,44.85 31.85,44.85 32.3,45.4 37.4,45.4 37.8,44.9 v37.8,42.9 | U$5.9 8.91,20.89 v9.4,20.4 | v38.7,46.8 SJ3.2
  Bottom 0.178: v19.8,36 20.2,36 v21.3,37.1 | v27.2,38.2 28.1,38.2 29.2,39.3 29.2,41.5 v31.35,44.85 | v9.4,20.4 9.4,21.2 10.2,22 10.2,24.3 9.3,25.2 9.3,26.4 9.5,26.6 9.5,33.8 9.6,33.9 16.1,33.9 16.2,34 v16.6,35.1 | v37.8,42.9 39.1,42.9 39.2,43 39.2,46.1 v38.7,46.8
HC05_RESET  (via drill 0.33 pad 0.25)  (1 unrouted)
  Top 0.178: 8.1,21.32 8.1,21.3 8.4,21 8.4,19.6 8.6,19.4 13.8,19.4 v13.8,20.1 | v33.3,24.95 v33.3,28.7 | SJ4.1 31.4,42.05 v31.4,40.8
  Bottom 0.178: v13.8,20.1 24.5,20 24.6,20.1 24.6,20.9 27.1,23.4 27.1,25 27.15,25.05 v33.3,24.95 | v31.4,40.8 31.8,40.4 31.8,40.3 31.9,40.2 32.8,40.2 33,40 33,29.4 33.3,29.1 v33.3,28.7
HC05_RESET_AVR  (via drill 0.33)
  Top 0.178: U$5.13 11.38,24.6 12.1,24.6 v12.1,24.8 | v34.5,38.8 34.5,39.82 34.62,39.94 R25.1 | v26.6,17.7 26.6,18.9 33.4,18.9 34.1,18.2 36.7,18.2 37.2,18.7 37.2,22.7 36,23.9 34.3,23.9 34.2,24 34.2,26 34.3,26.1 34.7,26.1 36.7,28.1 36.7,36.7 34.8,36.7 v34.2,37.3 | v15.8,18.1 15.8,20.3 v15.7,20.6
  Bottom 0.178: v12.1,24.8 12.4,24.8 12.4,22.4 16,22.4 16,20.8 v15.7,20.6 | v26.6,17.7 16.2,17.7 v15.8,18.1 | v34.2,37.3 34.2,38.1 34.5,38.4 v34.5,38.8
LED_GR
  Top 0.406: U2.11 26.93,28.27 27.4,27.8 27.4,26.25 R16.2
LED_RED
  Top 0.406: R15.2 26.33,24.27 25.8,24.8 25.8,27.1 25.7,27.2 24.8,27.2 24.6,27.4 23.08,27.4 U2.10
MISO
  Top 0.406: AVR_ISP.6 24.62,33.87 U2.16
MOSI
  Top 0.406: AVR_ISP.3 34.12,32.6 25.9,32.6 25.3,32 25.3,31.5 25.27,31.47 U2.15
N$1
  Top 0.406: D6.C 12.96,54.25
  Top 0.61: L1.2 7.42,54.59 C10.2 9.55,54.25 C9.1 12.96,54.25 | D6.C 13.02,54.4 | 15.47,46.57 IC2.3
  Top 0.813: 13.02,54.4 14.6,54.4 16.7,52.3 16.7,47.8 15.47,46.57
N$3
  Top 0.406: 7.28,49.12 R8.1 | R7.1 5.62,48.94 5.72,49.04 | 1.68,50.6 POWERSELECT.2 | 3.9,49.1 3.93,49.07
  Top 0.61: IC2.1 13.9,51.2 | 11.3,51.2 11.1,51 | 11.1,49.5 10.71,49.12
  Top 0.762: 13.9,51.2 11.3,51.2 | 11.1,51 11.1,49.5 | 10.71,49.12 D4.A 7.28,49.12 | 1.68,50.6 3.4,50.6 3.9,50.1 3.9,49.1 | 3.93,49.07 R7.1 | 5.72,49.04 R8.1
N$4
  Top 0.178: SJ1.1 35.08,44.75 R11.1
N$5  (via drill 0.33 pad 0.25)
  other vias: 21.46,39.5
N$6
  Top 0.178: U$1.4 8.09,5.15 8.09,6.52 7.35,7.26 6.32,7.26 6.09,7.49 6.09,10.22 6.42,10.55 8.68,10.55 9.33,11.2 IC1.5
N$7
  Top 0.178: U2.8 21.52,24.9 22.65,23.78
N$8
  Top 0.178: 20.95,22.08 20.95,24.05 20.7,24.3 20.7,25.15 U2.7
N$9  (via drill 0.33)
  Top 0.178: SJ4.2 32.65,42.2 v33.4,42.2
  Bottom 0.178: U3.11 36.06,31.3 33.7,31.3 33.6,31.4 33.6,40.4 33.4,40.6 v33.4,42.2
N$11
  Top 0.178: R12.2 26.54,44.35 D1.A
N$13
  Top 0.178: IC1.4 8.83,11.63 8.5,11.2 7.2,11.2 6.7,11 3.2,11 1.8,9.4 1.8,0.8 1.9,0.7 5.6,0.7 6.3,1.4 6.3,3.2 6.39,3.29 U$1.3
N$14  (via drill 0.33 pad 0.25)
  Top 0.178: 11.7,1.29 L3.1
  Top 0.406: 11.7,1.29 C1.2 | v15.75,4.06 15.75,1.66 C2.1
  Top 0.61: C2.1 15.75,1.26 15.17,1.26 14.84,1.29 C1.2
  Bottom 0.254: 15.62,4.57 15.75,4.45
  Bottom 0.406: U$3.VCC 11.43,8.48 11.43,4.95 11.81,4.57 15.62,4.57 | 15.75,4.45 v15.75,4.06
N$15  (via drill 0.33 pad 0.25)
  Top 0.178: v34.3,30.2 v31.5,30.1 | 34.7,42.3 36.61,42.3 | SJ1.2 36.61,42.3 | 36.61,42.3 36.5,42.19 36.5,38.1 31.8,38.1 31.2,38.8 v30.3,38.8
  Top 0.254: C21.1 11.9,39.6 v13.8,39.6 | v21.4,36.2 21.8,36.6 v27.6,36.6
  Top 0.406: L4.2 9.38,40.73 C19.1 C21.1
  Bottom 0.178: U3.12 35.74,30.2 v34.3,30.2 | v31.5,30.1 31.8,30.4 31.8,36.8 v30.3,38.8
  Bottom 0.254: v13.8,39.6 14.9,38.5 14.9,37.2 16.5,35.7 18.6,35.7 18.7,35.4 20.7,35.4 v21.4,36.2 | v27.6,36.6 27.8,36.8 31.8,36.8
N$17  (via drill 0.33 pad 0.25)
  Top 0.178: U2.24 15.92,35.52 16.1,35.7 18.7,35.7 19.5,36.5 v19.5,36.7 | v20.9,37.8 25.7,37.8 v26.7,38.8 | v28.5,39.9 32.6,39.9 32.6,39.92 R25.2
  Bottom 0.178: v19.5,36.7 19.9,36.8 v20.9,37.8 | v26.7,38.8 27.5,38.8 v28.5,39.9
N$18  (via drill 0.33 pad 0.25)
  Top 0.254: v13.34,6.86 v9.78,6.86
  Bottom 0.254: U$3.RXON | U$3.GPIO_0 9.3,7.4 9.37,7.4 v9.78,6.86 | 13.34,8.56 v13.34,6.86
  Bottom 0.406: U$3.RXON 13.34,8.56
N$19
  Bottom 0.254: U$3.TXON 15.2,8.71 15.2,10.3 15.1,10.4 8.2,10.4 7.3,9.5 U$3.GPIO_1
N$21  (via drill 0.5)
  Top 0.813: v19.32,6.81 v19.31,6.81 J3.P$3
  Bottom 0.813: U$3.ANT 19.32,8.6 v19.32,6.81
N$22  (via drill 0.33, 0.33 pad 0.25)
  Top 0.178: v25.36,45.31 25.39,45.34 29.84,45.34 30.09,45.09 | 30.09,45.09 31.24,43.94 31.24,43.5 32.93,43.5 R11.2 | SJ3.1 37.3,48.55 v37.3,48 | R2.1 30.09,44.04 30.09,45.09
  Bottom 0.178: U3.34 24.33,46.34 v25.36,45.31 25.65,45.6 33.1,45.6 34.9,47.3 37.3,47.3 v37.3,48
  Bottom 0.406: 23.24,46.2 U3.34
N$27
  Top 0.406: POWERSELECT.1 1.58,47.81 R17.1
N$28
  Top 0.254: IC1.9 13.54,13.93 R10.1
N$29
  Top 0.178: IC1.6 9.83,11.35 C18.1 C17.1 10.39,9.61 10.4,9.6
N$31
  Top 0.178: 28.92,24.08 28.92,21.26 LED1_RED.A
  Top 0.406: R15.1 28.92,24.08
N$32  (via drill 0.33)
  Top 0.178: v24.9,42 24.9,42.6 24.93,42.63 R12.1
  Bottom 0.178: U3.31 23.26,42 v24.9,42
N$34
  Top 0.406: R16.1 29.36,26.2 30.7,26.2 30.7,23.1 32.1,23.1 33,22.2 33,21.63 LED2_GREEN.A
N$35  (via drill 0.33 pad 0.25)
  Top 0.178: R1.2 10.13,30.8 v11,30.8 | U2.31 11.77,27.47 11.34,27.8 v10.95,27.8
  Bottom 0.178: v11,30.8 11,30.7 v10.95,27.8
N$38  (via drill 0.33 pad 0.25)
  Top 0.178: U2.26 16.16,31.47 v16.76,30.86 | v19.18,28.07 v19.18,26.67 | v19.68,21.21 19.68,17.02 v22.73,13.97 | v28.57,14.48 28.57,15.88 R20.2
  Bottom 0.178: v16.76,30.86 16.75,28.25 19.04,28.25 v19.18,28.07 | v19.18,26.67 19.18,21.72 v19.68,21.21 | v22.73,13.97 28.07,13.97 v28.57,14.48
N$43  (via drill 0.33 pad 0.25)
  Top 0.178: U2.30 14.4,28.3 v11.7,28.3 | v11.7,32.2 10.9,32.8 10.9,33.1 10.82,33.18 R19.2
  Bottom 0.178: v11.7,28.3 v11.7,32.2
PPM
  Top 0.178: TARANIS1.3 32.24,13.08 30.35,13.08 30.1,13.34 30.1,15.49 31.16,16.55 R20.1
  Top 0.406: 33.05,14.4 37.8,14.4 37.95,14.25 37.95,13.12 TARANIS1.4 37.97,12.52 37.3,11.85 32.25,11.85 32.2,11.9 32.2,13.04 TARANIS1.3
RESET  (via drill 0.33 pad 0.25)
  Top 0.178: 12.03,29.37 12.3,29.1 14.4,29.1 U2.29 14.46,29.18 18.3,29.18 19.8,30.6 v19.8,32.2 | 12.03,29.37 C22.2 | v21.4,32.2 24.2,35 v26,35 | 12.03,29.37 12.4,29.75 12.4,33.4 12.1,33.7 11.5,33.7 11.1,34.1 10.8,34.1 9.9,34.99 R14.2
  Top 0.254: AVR_ISP.2 27.96,28.79 26.96,29.79 26.57,29.79 26.4,29.96 v26.4,31
  Bottom 0.178: v19.8,32.2 v21.4,32.2 | v26,35 26.4,34.6 v26.4,31
RX  (via drill 0.33 pad 0.25)
  Top 0.178: IC1.26 6.3,14.4 4,14.4 3.6,14.85 3.6,26.85 4.85,28.1 6.5,28.1 | 6.5,28.1 9.8,28.1 10.1,27.8 10.1,27.1 9.7,26.7 9.7,26.5 9.27,26.07 U$5.18 | v6.1,28.5 6.5,28.1 | v6.1,30 6.1,31.7 6.8,32.4 8.08,32.4 8.2,32.52 R19.1
  Bottom 0.178: v6.1,30 v6.1,28.5
RX_3.3V  (via drill 0.33 pad 0.25)
  Top 0.178: v11,21.4 10.8,21.6 10.8,22.3 9.8,23.3 8.8,23.3 7.9,24.2 7.5,24.2 6.85,23.55 U$5.3 | v32.5,28.7 32.4,28.6 v32.4,24.25
  Bottom 0.178: v11,21.4 12.3,21.4 12.3,20.6 12.7,20.2 12.8,20.2 13.5,19.5 24.7,19.5 25.2,20 25.2,20.7 27.8,23.3 31.7,23.3 32.4,24 v32.4,24.25 | U3.1 34.54,46.34 34.5,46.3 34.5,45.5 32.5,43.5 32.5,41.9 30.6,41.9 30.5,41.8 30.5,39.9 30.7,39.7 32.3,39.7 32.5,39.5 v32.5,28.7
SCK  (via drill 0.33 pad 0.25)
  Top 0.406: U2.17 21.56,33.76 23.6,35.8 27.1,35.8 v27.7,35.2 | v27.5,30.9 29.26,30.9 AVR_ISP.4
  Bottom 0.406: v27.7,35.2 27.7,31.1 v27.5,30.9
TARANIS_BATT
  Top 0.254: TARANIS2.1 32.2,7.96
  Top 0.406: 32.2,7.96 32.2,7 32.5,6.7 36.95,6.7 37.97,7.72 TARANIS2.2 | TARANIS2.1 32.25,8.04 32.25,8.9 32.6,9.25 37.35,9.25 37.9,8.7 37.9,8.15 37.95,8.1
  Top 0.61: TARANIS2.1 29.52,8.03 SJ2.1
TX  (via drill 0.33 pad 0.25)
  Top 0.178: IC1.25 6.3,14.9 4.3,14.9 4.2,15 4.2,26.5 5.4,27.7 6.9,27.7 | 6.9,27.7 7.7,27.7 8,27.4 8,26.6 7.85,26.45 U$5.20 | R1.1 8.28,30.9 7.1,30.9 7,30.8 7,30.1 v6.9,30 | v6.9,27 6.9,27.7
  Bottom 0.178: v6.9,30 v6.9,27
TX_3.3V  (via drill 0.33 pad 0.25)
  Top 0.178: U$5.1 6.4,25.36 6.4,25.7 v6.1,26 | v38.5,44.7 38.5,41.8 37.9,41.8 37.2,41.1 37.2,40.4 36.93,40.13 36.93,38.35 37.1,38.22 37.1,27.8 34.9,25.6 v34.9,24.65
  Bottom 0.178: v38.5,44.7 38.36,44.84 U3.2 | v34.9,24.65 34.55,24.65 32.4,22.5 27.9,22.5 26.3,20.9 26.3,20.2 25,18.9 6.7,19 6.3,19 6.3,23.4 6.9,24 6.9,25.6 6.5,25.6 v6.1,26
VBAT  (via drill 0.33 pad 0.25)
  Top 0.61: C6.1 5.08,53.11 L1.1 6.86,53.07 v6.86,51.94 | SJ2.2 28.98,3.23 JP1.2 | v37.21,26.8 37.41,27.08 37.77,27.56 37.77,39.24 37.72,39.5 37.72,40.13 38.86,41.27 38.99,41.27 39.24,41.53 39.24,45.34 38.61,45.97 26.29,45.97 26.04,46.23 25.02,46.23 24.59,46.05 21.92,46.05 21.84,46.2 21.84,51.82 v21.72,51.94
  Bottom 0.61: v21.72,51.94 v6.86,51.94
  Bottom 0.762: v37.21,26.8 37.21,16.89 38.73,16.26 39.98,14.66 39.94,2.39 38.8,1.08 30.15,1.1 JP1.2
